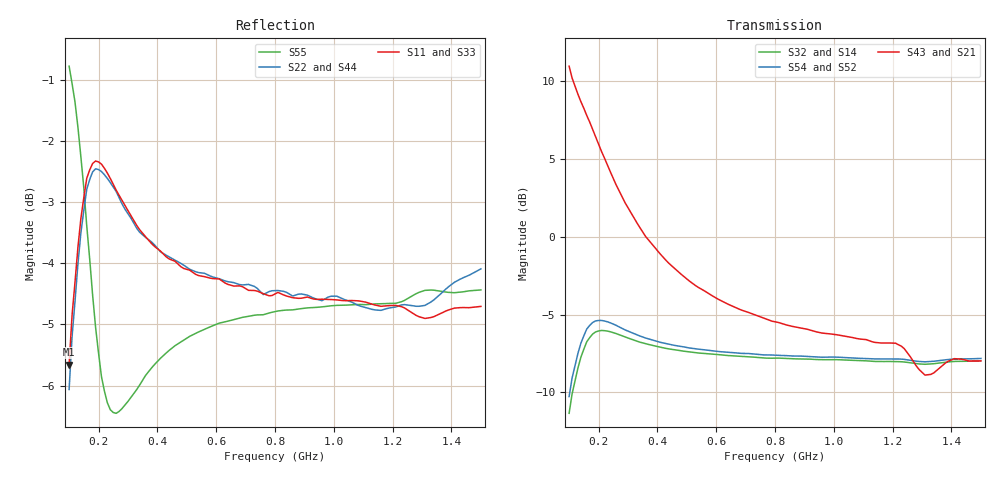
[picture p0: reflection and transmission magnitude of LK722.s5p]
! Date: Fri Jan 15 13:14:26 1999
!  POLYFET RF DEVICES
!  LP722/LK722
!  12.5Vdc		400ma
!AWR Design Environment (2053) Wed Feb 04 14:54:21 2004
!freq-unit  param-type  data-format  keyword  impedance-ohms
# MHz  S  MA  R  50
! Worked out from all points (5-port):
!   141 points, 100 MHz to 1.5 GHz, reference 50 ohm
!   strongest paths, dB at 100 MHz, 450 MHz, 800 MHz, 1.15 GHz, 1.5 GHz:
!     S43: 11.0, -1.9, -5.5, -6.8, -8.0
!     S21: 11.0, -1.9, -5.5, -6.8, -8.0
!     S54: -10.3, -6.9, -7.6, -7.9, -7.8
!     S52: -10.3, -6.9, -7.6, -7.9, -7.8
!     S32: -11.4, -7.2, -7.8, -8.0, -8.0
!     S14: -11.4, -7.2, -7.8, -8.0, -8.0
!   lowest |S11| = -5.7 dB at 100 MHz (marker M1), VSWR 3.18, Z = 29.2 - j41.9 ohm
!   |S11| at or under -10 dB: nowhere
